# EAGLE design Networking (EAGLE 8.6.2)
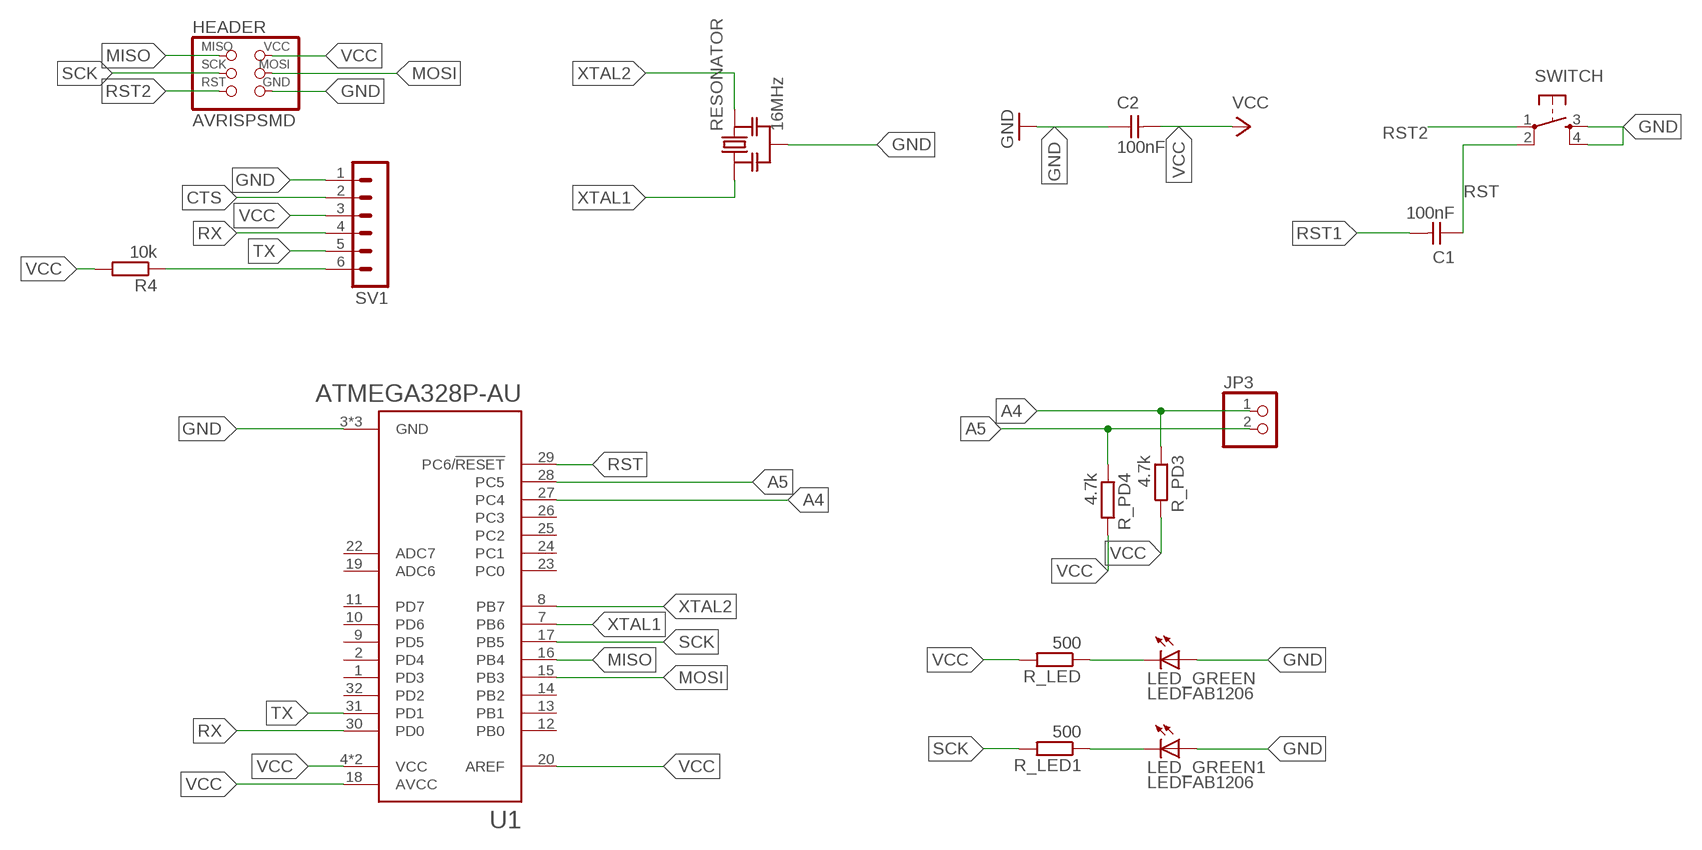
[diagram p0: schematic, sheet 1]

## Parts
C1  100nF  CAP-UNPOLARIZEDFAB  [C1206FAB]
C2  100nF  CAP-UNPOLARIZEDFAB  [C1206FAB]
HEADER  AVRISPSMD  [2X03SMD]
JP3  PINHD-1X2  [1X02]
LED_GREEN  LEDFAB1206  [LED1206FAB]
LED_GREEN1  LEDFAB1206  [LED1206FAB]
R4  10k  R-EU_R1206  [R1206]
R_LED  500  R-EU_R1206  [R1206]
R_LED1  500  R-EU_R1206  [R1206]
R_PD3  4.7k  R-EU_R1206  [R1206]
R_PD4  4.7k  R-EU_R1206  [R1206]
RESONATOR  16MHz  RESONATOR-MURATACSTCR_G  [RESONATOR_MURATA3]
SV1  MA06-1  [MA06-1]
SWITCH  6MM_SWITCH6MM_SWITCH  [6MM_SWITCH]
U1  ATMEGA328P-AU  [QFP80P900X900X120-32N]

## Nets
A4: JP3.1 R_PD3.1 U1.27(PC4)
A5: JP3.2 R_PD4.1 U1.28(PC5)
CTS: SV1.2
GND: C2.1 HEADER.6(GND) LED_GREEN1.1(A) LED_GREEN.1(A) RESONATOR.2 SV1.1 SWITCH.3(S) SWITCH.4(S1) U1.3(GND) U1.5(GND) U1.21(GND)
MISO: HEADER.1(MISO) U1.16(PB4)
MOSI: HEADER.4(MOSI) U1.15(PB3)
N$1: LED_GREEN1.2(C) R_LED1.1
N$21: LED_GREEN.2(C) R_LED.1
RST: C1.1 SWITCH.2(P1) U1.29(PC6/!RESET)
RST1: C1.2 R4.1 SV1.6
RST2: HEADER.5(RST) SWITCH.1(P)
RX: SV1.4 U1.30(PD0)
SCK: HEADER.3(SCK) R_LED1.2 U1.17(PB5)
TX: SV1.5 U1.31(PD1)
VCC: C2.2 HEADER.2(VCC) R4.2 R_LED.2 R_PD3.2 R_PD4.2 SV1.3 U1.4(VCC) U1.6(VCC) U1.18(AVCC) U1.20(AREF)
XTAL1: RESONATOR.1 U1.7(PB6)
XTAL2: RESONATOR.3 U1.8(PB7)
Unconnected: U1.1(PD3) U1.2(PD4) U1.9(PD5) U1.10(PD6) U1.11(PD7) U1.12(PB0) U1.13(PB1) U1.14(PB2) U1.19(ADC6) U1.22(ADC7) U1.23(PC0) U1.24(PC1) U1.25(PC2) U1.26(PC3) U1.32(PD2)

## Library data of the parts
C1 C2 = fab:CAP-UNPOLARIZED
HEADER = fab:AVRISP
JP3 = pinhead:PINHD-1X2: PIN HEADER
LED_GREEN LED_GREEN1 = fab:LED: LED
R4 R_LED R_LED1 R_PD3 R_PD4 = resistor:R-EU_: RESISTOR, European symbol
RESONATOR = m-pad-2.1:RESONATOR-MURATA: Murata ceramic Resonator "ceralock" CSTCE series with built in load capacitance +- 0.5% tolerance 12.51MHz to 19.99MHz 16MHz murata part#: CSTCE16M0V53-R0 16MHz digikey part#: 490-1198-1-ND $1.33 each
SV1 = con-lstb:MA06-1: PIN HEADER; OC_FARNELL: unknown; OC_NEWARK: unknown
SWITCH = fab:6MM_SWITCH: OMRON SWITCH
U1 = ATMEGA328P-AU:ATMEGA328P-AU: ATmega Series 20 MHz 32 KB Flash 2 KB SRAM 8-Bit Microcontroller - TQFP-32; AVAILABILITY: Good; DESCRIPTION: ATmega Series 20 MHz 32 KB Flash 2 KB SRAM 8-Bit Microcontroller - TQFP-32; MF: Atmel; MP: ATMEGA328P-AU; PACKAGE: TQFP-32 Atmel; PRICE: 2.38 USD

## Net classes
0 default: clearance 0.205 mm

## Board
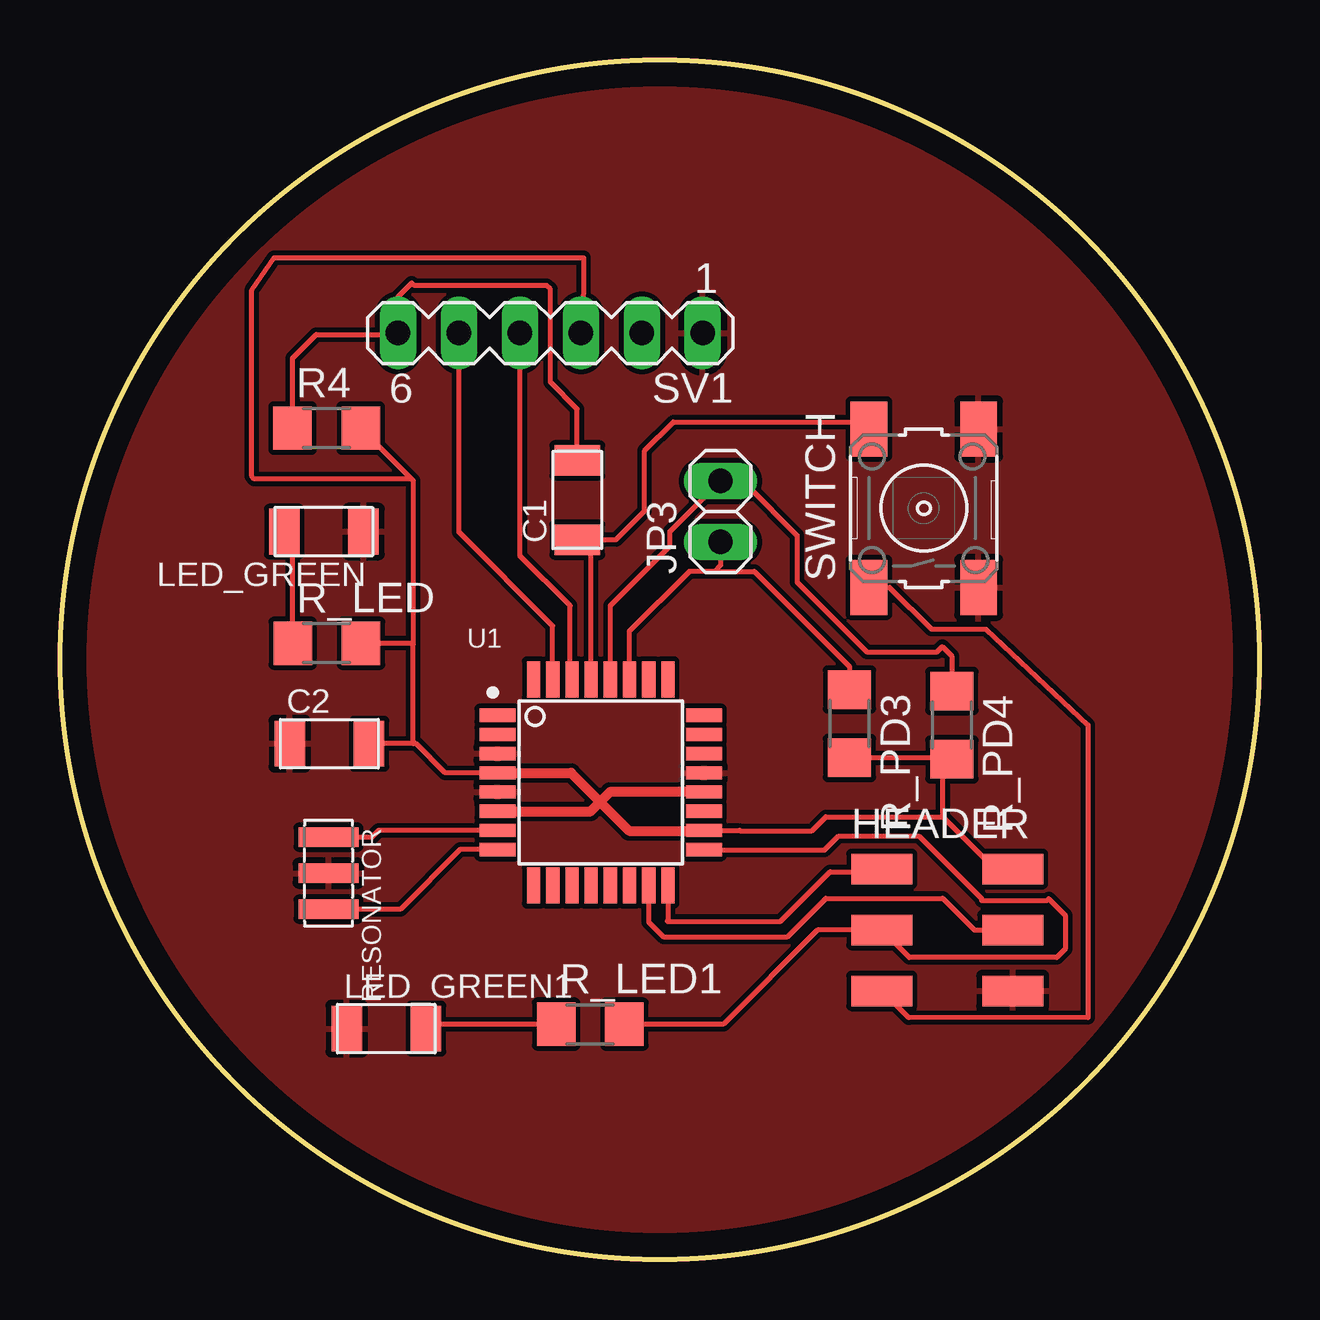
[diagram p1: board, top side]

Size 50 x 50 mm. Coordinates in mm from the lower left corner, seen from the top.
Outline: circle at 25,25 radius 25
Copper layers (1*16): Top 0.035mm / dielectric 1.5mm / Bottom 0.035mm
Design rules "default *": minimum track width 6mil, minimum drill 0.35mm, track to track 8mil, track to pad 8mil, pad to pad 8mil, via to via 8mil, smd to smd 8mil, copper to edge 40mil, drill to drill 8mil, minimum pad ring 10mil, minimum via ring 8mil, stop-mask expansion 4mil, vias tented up to drill 0mil, thermal gap 10mil

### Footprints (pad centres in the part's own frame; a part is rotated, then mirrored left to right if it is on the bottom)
C1206FAB = smd 1.27 x 1.905: 1 -1.651,0; 2 1.651,0
2X03SMD = smd 2.54 x 1.27: 1 -2.54,2.54; 2 2.92,2.54; 3 -2.54,0; 4 2.92,0; 5 -2.54,-2.54; 6 2.92,-2.54
1X02 = drill 1.016 long: 1 -1.27,0; 2 1.27,0
LED1206FAB = smd 1.27 x 1.905: 1 -1.651,0; 2 1.651,0
R1206 = smd 1.6 x 1.803: 1 -1.422,0; 2 1.422,0
RESONATOR_MURATA3 = smd 0.8 x 2.5: 1 -1.5,0; 2 0,0; 3 1.5,0
MA06-1 = drill 1.016 long: 1 -6.35,0; 2 -3.81,0; 3 -1.27,0; 4 1.27,0; 5 3.81,0; 6 6.35,0
6MM_SWITCH = smd 2.286 x 1.524: 1 -3.302,2.286; 2 3.302,2.286; 3 -3.302,-2.286; 4 3.302,-2.286
QFP80P900X900X120-32N = smd 1.5 x 0.55: 1 -4.3,2.8; 2 -4.3,2; 3 -4.3,1.2; 4 -4.3,0.4; 5 -4.3,-0.4; 6 -4.3,-1.2; 7 -4.3,-2; 8 -4.3,-2.8; 17 4.3,-2.8; 18 4.3,-2; 19 4.3,-1.2; 20 4.3,-0.4; 21 4.3,0.4; 22 4.3,1.2; 23 4.3,2; 24 4.3,2.8 | smd 0.55 x 1.5: 9 -2.8,-4.3; 10 -2,-4.3; 11 -1.2,-4.3; 12 -0.4,-4.3; 13 0.4,-4.3; 14 1.2,-4.3; 15 2,-4.3; 16 2.8,-4.3; 25 2.8,4.3; 26 2,4.3; 27 1.2,4.3; 28 0.4,4.3; 29 -0.4,4.3; 30 -1.2,4.3; 31 -2,4.3; 32 -2.8,4.3

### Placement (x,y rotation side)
C1  21.56,31.66 90 top
C2  11.23,21.5 0 top
HEADER  36.79,13.74 0 top
JP3  27.53,31.18 90 top
LED_GREEN  11,30.34 180 top
LED_GREEN1  13.6,9.62 0 top
R4  11.11,34.66 0 top
R_LED  11.13,25.69 0 top
R_LED1  22.1,9.81 0 top
R_PD3  32.91,22.33 270 top
R_PD4  37.17,22.27 270 top
RESONATOR  11.19,16.1 270 top
SV1  20.44,38.62 180 top
SWITCH  36.01,31.32 90 top
U1  22.54,19.89 0 top

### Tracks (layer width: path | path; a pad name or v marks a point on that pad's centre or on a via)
A4
  Top 0.2: U1.27 23.74,26.19 26.23,28.69 27.27,28.69 | JP3.1 27.53,28.95 27.27,28.69 | 27.27,28.69 28.94,28.69 32.91,24.72 R_PD3.1
A5
  Top 0.2: U1.28 22.94,27.26 25.43,29.75 25.43,30.35 JP3.2 27.73,32.26 28.65,32.26 30.73,30.18 30.73,28.23 33.63,25.33 36.56,25.33 36.77,25.54 37.17,25.15 R_PD4.1
GND
  pour Top: -43.5,77.04 -43.5,-58.85 -42.23,-60.12 73.34,-60.12 79.69,-53.77 79.69,78.31 69.53,88.47 -32.07,88.47
MISO
  Top 0.2: U1.16 25.34,14.13 25.31,14.1 30.04,14.1 32.1,16.16 34.14,16.16 HEADER.1
MOSI
  Top 0.2: U1.15 24.54,14.06 25.15,13.45 30.31,13.45 31.92,15.06 36.79,15.06 38.12,13.74 HEADER.4
N$1
  Top 0.2: R_LED1.1 15.44,9.81 LED_GREEN1.2
N$21
  Top 0.2: R_LED.1 9.71,29.98 LED_GREEN.2
RST
  Top 0.2: C1.1 21.6,30.01 | 21.6,30.01 23.17,30.01 24.37,31.2 24.37,33.71 25.56,34.91 33.43,34.91 SWITCH.2 | U1.29 22.14,29.47 21.6,30.01
RST1
  Top 0.2: R4.1 9.69,37.57 10.68,38.56 14.03,38.56 SV1.6 14.09,40.13 14.67,40.7 14.76,40.6 20.28,40.6 20.44,40.45 20.44,36.58 21.56,35.46 C1.2
RST2
  Top 0.2: SWITCH.1 34.58,28.01 36.32,26.27 38.6,26.27 42.85,22.28 42.85,10.09 35.38,10.07 HEADER.5
RX
  Top 0.2: U1.30 21.26,24.26 21.26,27.25 19.16,29.35 19.17,29.36 SV1.4
SCK
  Top 0.2: U1.17 26.86,17.06 31.87,17.06 32.45,17.65 35.79,17.65 38.42,15.02 38.42,14.96 41.13,14.96 41.21,15.04 41.9,14.35 41.9,12.94 41.55,12.59 35.4,12.59 HEADER.3 31.58,13.74 27.65,9.81 R_LED1.2
TX
  Top 0.2: U1.31 20.54,26.41 16.63,30.32 SV1.5
VCC
  Top 0.2: U1.18 28.33,17.89 28.35,17.87 31.34,17.87 31.92,18.46 36.79,18.46 | 36.79,18.46 38.98,16.28 HEADER.2 | U1.4 16.06,20.29 14.84,21.5 14.72,21.5 | 14.72,21.5 C2.2 | 14.72,21.5 14.72,25.64 | 14.72,25.64 14.72,32.46 14.65,32.54 | R_LED.2 14.68,25.69 14.72,25.64 | R4.2 14.65,32.54 | R_PD3.2 37.11,20.91 R_PD4.2 36.79,20.47 36.79,18.46 | 14.65,32.54 8.1,32.54 7.99,32.65 7.99,40.41 8.93,41.75 21.83,41.75 21.79,38.7 SV1.3
  Top 0.406: U1.4 21.31,20.29 22.51,19.08 | 22.51,19.08 23.73,17.87 26.82,17.87 U1.18 | U1.6 22.12,18.69 22.51,19.08 | U1.20 22.92,19.49 22.51,19.08
XTAL1
  Top 0.2: U1.7 13.29,17.89 13,17.59 11.2,17.59 RESONATOR.1
XTAL2
  Top 0.2: U1.8 16.67,17.09 14.19,14.6 RESONATOR.3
